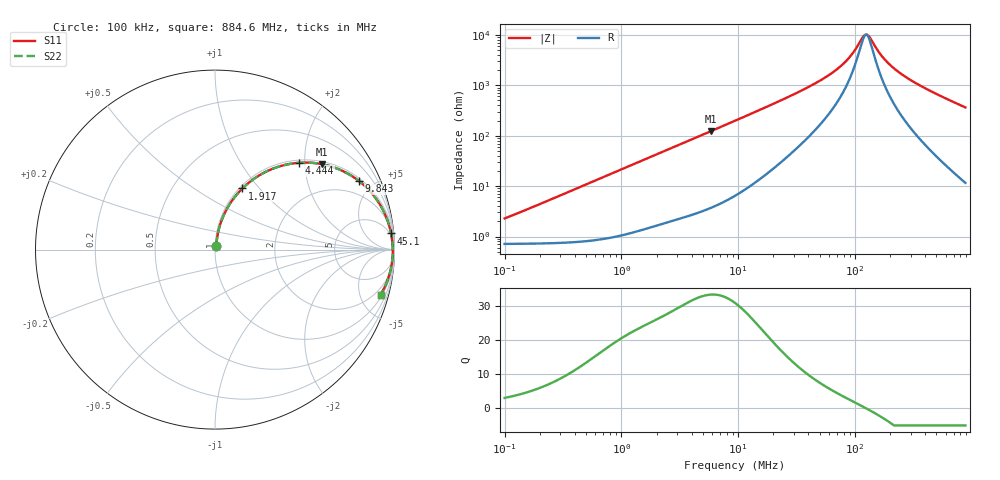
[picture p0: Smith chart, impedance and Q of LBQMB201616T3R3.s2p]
! LBQMB201616T3R3  S-PARAMETER MODEL  ( General Type )
! Model Generated by TAIYO YUDEN Corporation (http://www.ty-top.com)
! Version 1.0
! TAIYO YUDEN Control No. 191025NI43SB-FBB
! Copyright(c) 2019 TAIYO YUDEN CO.,LTD. All Rights Reserved.
! Product Description (link to TY-COMPAS)
! https://ds.yuden.co.jp/TYCOMPAS/or/detail?pn=LBQMB201616T3R3J&u=M
! Products Name : Inductors
! Characteristics :
!  Inductance : 3.3 uH , SRF(min) : 48 MHz , DC Resistance(max) : 0.884 Ohm , Rated Current : 290 mA
!  Case Size : 2.0 x 1.6 / 0.079 x 0.063 [mm/inch] , Thickness : 1.6 / 0.063 [mm/inch]
!  (Conditions: Temperature = 25 degC , DC Bias Current/Voltage = 0A / 0V)
! External Node Assignments :
!  1  o---GGG---o  2
! GND o---------o GND
! Frequency Range : 0.1MHz  -  884.637303MHz  [ 402 STEP ]
# MHz S RI R 50
! Freq[MHz].  S11 Real  S11 Imag  S21 Real  S21 Imag  S12 Real  S12 Imag  S22 Real  S22 Imag
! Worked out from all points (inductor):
!   401 points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, 100 kHz to 884.6 MHz, reference 50 ohm
!   read as one part in series: L = 3.45 uH near 104.6 kHz
!   highest Q = 33.2 at 5.837 MHz (marker M1), where L = 3.34 uH
!   self-resonance near 122.6 MHz
!   S11 on the Smith chart (normalised r, x): 100 kHz: 1.01, +0.04; 1.917 MHz: 1.03, +0.82; 4.444 MHz: 1.06, +1.87; 9.843 MHz: 1.14, +4.14; 45.1 MHz: 4, +21; 884.6 MHz: 1.23, -7.27
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0.1  0.00753 0.0214  0.9925 -0.0214  0.9925 -0.0214  0.00753 0.0214
0.45823  0.0173 0.0965  0.9827 -0.0965  0.9827 -0.0965  0.0173 0.0965
1.062084  0.0586 0.2123  0.9414 -0.2123  0.9414 -0.2123  0.0586 0.2123
1.917338  0.1524 0.3404  0.8476 -0.3404  0.8476 -0.3404  0.1524 0.3404
2.099744  0.1754 0.3618  0.8246 -0.3618  0.8246 -0.3618  0.1754 0.3618
4.444005  0.4676 0.4837  0.5324 -0.4837  0.5324 -0.4837  0.4676 0.4837
5.836835  0.5979 0.4755  0.4021 -0.4755  0.4021 -0.4755  0.5979 0.4755
9.405516  0.789 0.3921  0.211 -0.3921  0.211 -0.3921  0.789 0.3921
9.84275  0.8031 0.3815  0.1969 -0.3815  0.1969 -0.3815  0.8031 0.3815
18.17704  0.9277 0.2362  0.0723 -0.2362  0.0723 -0.2362  0.9277 0.2362
43.09886  0.98 0.0951  0.02 -0.0951  0.02 -0.0951  0.98 0.0951
45.1024  0.981 0.0898  0.019 -0.0898  0.019 -0.0898  0.981 0.0898
61.99211  0.9862 0.0571  0.0138 -0.0571  0.0138 -0.0571  0.9862 0.0571
79.59256  0.9885 0.0352  0.0115 -0.0352  0.0115 -0.0352  0.9885 0.0352
93.31272  0.9894 0.0224  0.0106 -0.0224  0.0106 -0.0224  0.9894 0.0224
122.5586  0.9903 0.00148  0.00973 -0.00148  0.00973 -0.00148  0.9903 0.00148
134.2182  0.9904 -0.00546  0.00964 0.00546  0.00964 0.00546  0.9904 -0.00546
164.6697  0.9902 -0.0214  0.0098 0.0214  0.0098 0.0214  0.9902 -0.0214
197.4918  0.9896 -0.0364  0.0104 0.0364  0.0104 0.0364  0.9896 -0.0364
253.5625  0.9876 -0.0591  0.0124 0.0591  0.0124 0.0591  0.9876 -0.0591
348.5153  0.9825 -0.0934  0.0175 0.0934  0.0175 0.0934  0.9825 -0.0934
884.6373  0.9228 -0.2514  0.0772 0.2514  0.0772 0.2514  0.9228 -0.2514
